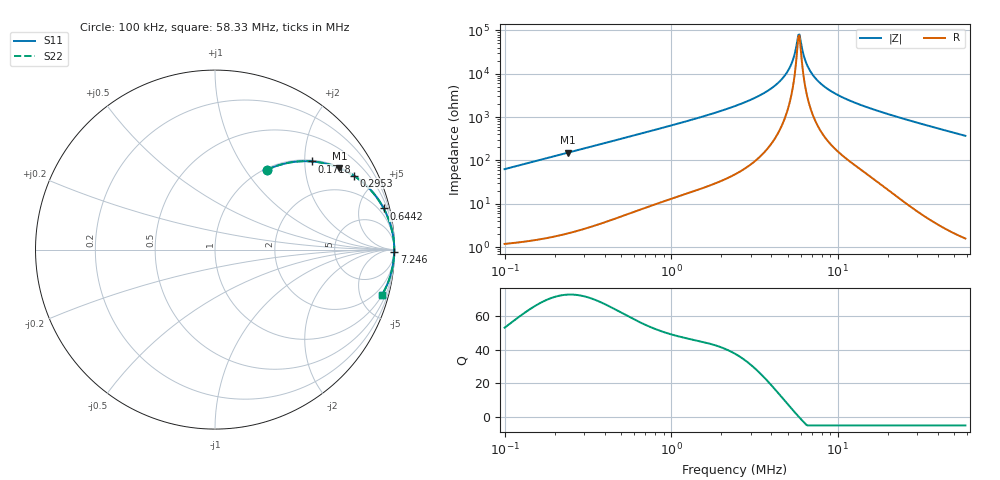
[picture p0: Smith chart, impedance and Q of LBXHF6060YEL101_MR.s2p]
! LBXHF6060YEL101_MR  S-PARAMETER MODEL  ( General Type )
! Model Generated by TAIYO YUDEN Corporation (http://www.ty-top.com)
! Version 1.0
! TAIYO YUDEN Control No. 200120NI43SB-FBB
! Copyright(c) 2020 TAIYO YUDEN CO.,LTD. All Rights Reserved.
! Product Description (link to TY-COMPAS)
! https://ds.yuden.co.jp/TYCOMPAS/or/detail?pn=LBXHF6060YEL101MMR&u=M
! Products Name : Inductors
! Characteristics :
!  Inductance : 100 uH , SRF(min) : 4.0 MHz , DC Resistance(max) : 0.6 Ohm
!  Rated Current : Saturation :1050 mA , Temp Rise : 550 mA
!  Case Size : 6.0 x 6.0 / 0.236 x 0.236 [mm/inch] , Thickness : 4.5 / 0.177 [mm/inch]
!  (Conditions: Temperature = 25 degC , DC Bias Current/Voltage = 0A / 0V)
! External Node Assignments :
!  1  o---GGG---o  2
! GND o---------o GND
! Frequency Range : 0.1MHz  -  58.334721MHz  [ 402 STEP ]
# MHz S RI R 50
! Freq[MHz].  S11 Real  S11 Imag  S21 Real  S21 Imag  S12 Real  S12 Imag  S22 Real  S22 Imag
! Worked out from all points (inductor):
!   401 points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, 100 kHz to 58.33 MHz, reference 50 ohm
!   read as one part in series: L = 100 uH near 103.2 kHz
!   highest Q = 72.6 at 240.1 kHz (marker M1), where L = 100 uH
!   self-resonance near 5.798 MHz
!   S11 on the Smith chart (normalised r, x): 100 kHz: 1.02, +1.26; 171.8 kHz: 1.03, +2.17; 295.3 kHz: 1.05, +3.72; 644.2 kHz: 1.14, +8.15; 7.246 MHz: open; 58.33 MHz: 1.03, -7.40
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0.1  0.2885 0.4437  0.7115 -0.4437  0.7115 -0.4437  0.2885 0.4437
0.171832  0.5393 0.4912  0.4607 -0.4912  0.4607 -0.4912  0.5393 0.4912
0.240057  0.6935 0.4542  0.3065 -0.4542  0.3065 -0.4542  0.6935 0.4542
0.290598  0.7672 0.4157  0.2328 -0.4157  0.2328 -0.4157  0.7672 0.4157
0.295262  0.7728 0.4121  0.2272 -0.4121  0.2272 -0.4121  0.7728 0.4121
0.644219  0.9397 0.2294  0.0603 -0.2294  0.0603 -0.2294  0.9397 0.2294
0.844473  0.9633 0.1785  0.0367 -0.1785  0.0367 -0.1785  0.9633 0.1785
2.454022  0.9956 0.0542  0.00441 -0.0542  0.00441 -0.0542  0.9956 0.0542
3.596119  0.998 0.028  0.00197 -0.028  0.00197 -0.028  0.998 0.028
4.566214  0.9987 0.0139  0.00133 -0.0139  0.00133 -0.0139  0.9987 0.0139
5.186505  0.9988 0.00667  0.00119 -0.00667  0.00119 -0.00667  0.9988 0.00667
5.440255  0.9988 0.00402  0.00117 -0.00402  0.00117 -0.00402  0.9988 0.00402
5.70642  0.9988 0.00137  0.00117 -0.00137  0.00117 -0.00137  0.9988 0.00137
5.798004  0.9988 0.000488  0.00118 -0.000488  0.00118 -0.000488  0.9988 0.000488
5.985607  0.9988 -0.00127  0.00119 0.00127  0.00119 0.00127  0.9988 -0.00127
6.379218  0.9988 -0.0048  0.00124 0.0048  0.00124 0.0048  0.9988 -0.0048
7.018695  0.9986 -0.0101  0.00137 0.0101  0.00137 0.0101  0.9986 -0.0101
7.245794  0.9986 -0.0119  0.00143 0.0119  0.00143 0.0119  0.9986 -0.0119
8.362177  0.9982 -0.0201  0.0018 0.0201  0.0018 0.0201  0.9982 -0.0201
10.28518  0.9974 -0.0326  0.00263 0.0326  0.00263 0.0326  0.9974 -0.0326
20.39619  0.991 -0.0863  0.00902 0.0863  0.00902 0.0863  0.991 -0.0863
58.33472  0.931 -0.2514  0.069 0.2514  0.069 0.2514  0.931 -0.2514
